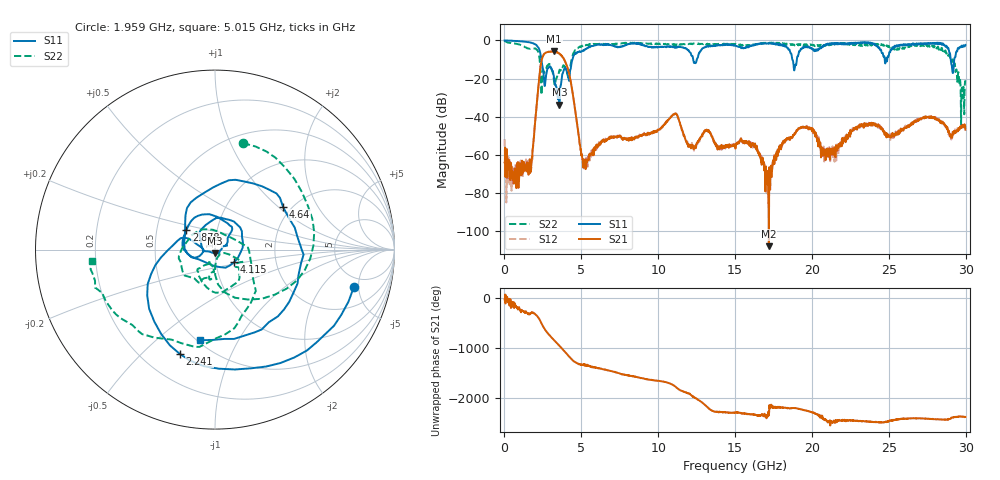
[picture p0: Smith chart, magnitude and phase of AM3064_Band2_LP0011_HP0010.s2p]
# Hz S DB R 50.0
!freq dBS11 angS11 dBS21 angS21 dBS12 angS12 dBS22 angS22
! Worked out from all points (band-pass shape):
!   1600 points, 10 MHz to 29.98 GHz, reference 50 ohm
!   highest |S21| = -5.75 dB at 3.234 GHz (marker M1); lowest = -108.0 dB at 17.2 GHz (marker M2)
!   |S21| within 3 dB of the highest: 2.474 GHz to 3.787 GHz (1.314 GHz wide, 42 % of centre)
!   lowest |S11| = -33.8 dB at 3.571 GHz (marker M3), VSWR 1.04, Z = 49.8 - j2.04 ohm
!   |S11| at or under -10 dB: 2.403 GHz to 4.425 GHz (2.022 GHz wide, 59.2 % of centre); 18.73 GHz to 19.02 GHz (294.7 MHz wide, 1.56 % of centre); 29.03 GHz to 29.26 GHz (228.3 MHz wide, 0.783 % of centre)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
!   |S22| runs from -45.2 to -0.2 dB; largest |S21 - S12| = 0.018
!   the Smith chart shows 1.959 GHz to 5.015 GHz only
!   S11 on the Smith chart (normalised r, x): 1.959 GHz: 3.73, -4.39; 2.241 GHz: 0.35, -0.66; 2.878 GHz: 0.71, +0.16; 4.115 GHz: 1.23, -0.17; 4.64 GHz: 1.81, +1.07; 5.015 GHz: 0.52, -0.71
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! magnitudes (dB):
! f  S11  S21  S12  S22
! 10 MHz  0.0  -64.1  -51.8  -0.2
! 441.1 MHz  -0.2  -66.6  -66.0  -1.4
! 1.584 GHz  -1.0  -68.7  -68.7  -4.3
! 1.959 GHz  -1.9  -46.0  -46.5  -4.2
! 2.241 GHz  -4.2  -21.4  -21.3  -7.6
! 2.878 GHz  -14.3  -5.9  -6.0  -12.5
! 3.234 GHz  -20.5  -5.8  -6.0  -22.3
! 3.571 GHz  -33.8  -7.0  -6.9  -15.6
! 4.115 GHz  -17.8  -14.8  -14.6  -18.4
! 4.64 GHz  -7.0  -38.8  -38.7  -5.1
! 5.015 GHz  -5.8  -59.5  -59.6  -3.3
! 10 GHz  -3.5  -47.1  -47.2  -1.8
! 15 GHz  -2.6  -55.4  -55.4  -1.9
! 16.32 GHz  -2.3  -55.3  -55.1  -2.0
! 17.2 GHz  -1.6  -108.0  -81.0  -1.6
! 18.04 GHz  -2.4  -54.5  -55.3  -2.0
! 19.99 GHz  -4.1  -47.0  -46.6  -2.2
! 20.95 GHz  -2.4  -60.6  -57.7  -2.2
! 25 GHz  -8.0  -50.6  -51.0  -2.8
! 28.56 GHz  -2.1  -43.4  -43.5  -4.7
! 29.18 GHz  -17.1  -48.0  -49.6  -10.2
! 29.98 GHz  -2.4  -46.8  -44.9  -21.5
